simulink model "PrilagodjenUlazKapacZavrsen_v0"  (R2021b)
settings: Solver=VariableStepAuto  StartTime=0.0  StopTime=200e-09  MaxStep=0.1e-09  RelTol=1e-3
libraries: fl_lib x9, nesl_utility x5, simulink x1, ee_lib x1

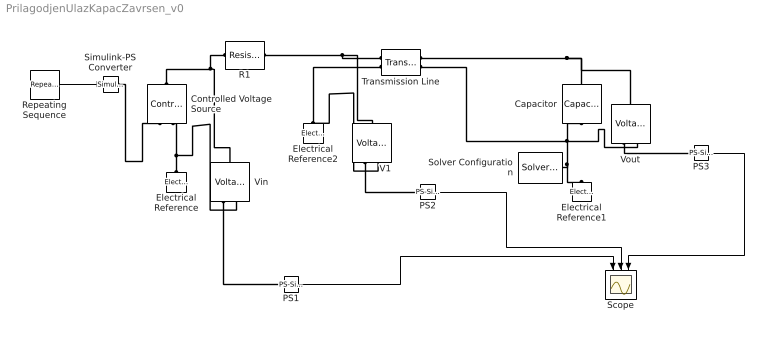
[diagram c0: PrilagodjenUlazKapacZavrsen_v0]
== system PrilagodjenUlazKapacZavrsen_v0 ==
  Capacitor : fl_lib/Electrical/Electrical Elements/Capacitor  c=200 pF  r=1e-6 Ohm  g=0 1/Ohm  i_specify=off  i_priority=None  i=0 A  i_nominal_specify=off  i_nominal_unit=A  i_nominal_value=1  v_specify=off  v_priority=None  v=0 V  v_nominal_specify=off  v_nominal_unit=V  v_nominal_value=1  vc_specify=off  vc_priority=High  vc=0 V  vc_nominal_specify=off  vc_nominal_unit=V  vc_nominal_value=1
  Controlled Voltage Source : fl_lib/Electrical/Electrical Sources/Controlled Voltage Source
  Electrical Reference : fl_lib/Electrical/Electrical Elements/Electrical Reference
  Electrical Reference1 : fl_lib/Electrical/Electrical Elements/Electrical Reference
  Electrical Reference2 : fl_lib/Electrical/Electrical Elements/Electrical Reference
  PS1 : nesl_utility/PS-Simulink Converter  PhysicalDomain=network_engine_domain  SubClassName=ps_output  LeftPortType=input  RightPortType=output  PseudoPeriodic=off  Frequencies=[]  Unit=inherit  AffineConversion=off
  PS2 : nesl_utility/PS-Simulink Converter  PhysicalDomain=network_engine_domain  SubClassName=ps_output  LeftPortType=input  RightPortType=output  PseudoPeriodic=off  Frequencies=[]  Unit=inherit  AffineConversion=off
  PS3 : nesl_utility/PS-Simulink Converter  PhysicalDomain=network_engine_domain  SubClassName=ps_output  LeftPortType=input  RightPortType=output  PseudoPeriodic=off  Frequencies=[]  Unit=inherit  AffineConversion=off
  R1 : fl_lib/Electrical/Electrical Elements/Resistor  R=50 Ohm  i_specify=off  i_priority=None  i=0 A  i_nominal_specify=off  i_nominal_unit=A  i_nominal_value=1  v_specify=off  v_priority=None  v=0 V  v_nominal_specify=off  v_nominal_unit=V  v_nominal_value=1
  Repeating Sequence : simulink/Sources/Repeating Sequence  rep_seq_t=[0 1 20 21 300]*1e-9  rep_seq_y=[0 1 1 0 0]
  Scope : Scope  NumInputPorts=3
  Simulink-PS Converter : nesl_utility/Simulink-PS Converter  PhysicalDomain=network_engine_domain  SubClassName=ps_input  LeftPortType=input  RightPortType=output  PseudoPeriodic=off  Frequencies=[]  NoiseDistribution=none  NoiseParameters=[]  Unit=1  AffineConversion=off  FilteringAndDerivatives=provide  SimscapeFilterOrder=1  InputFilterTimeConstant=0.001  UdotUserProvided=0
  Solver Configuration : nesl_utility/Solver Configuration  PhysicalDomain=network_engine_domain  SubClassName=solver  LeftPortType=input  RightPortType=generic  Tones=[]  Harmonics=[]  SimulateNoise=off  Profile=off  UseLocalSampling=off  EnableSwitchedLinearOptims=on  FrequencyDomain=off  UseCCode=off  RelTol=0.001  AbsTol=1e-06  MinStep=1e-09  ToWorkspace=off  RevertToSquareIcSolve=off  NumHomotopyIterations=100  PhasorMode=off  PhasorModeNumHarmonics=1  DoDC=off  ResidualTolerance=1e-09  UseLocalSolver=off  LocalSolverChoice=NE_BACKWARD_EULER_ADVANCER  LocalSolverSampleTime=0.001  DoFixedCost=off  MaxNonlinIter=3  MaxModeIter=2  ComputeImpulses=off  ImpulseIterations=2  LinearAlgebra=auto  EquationFormulation=NE_TIME_EF  DelaysMemoryBudget=1024  AutomaticFiltering=on  FilteringTimeConstant=0.001  PartitionStorageMethod=AS_NEEDED  PartitionMemoryBudget=1024  PartitionMethod=ROBUST
  Transmission Line : ee_lib/Passive/Lines/Transmission Line  model_type=1  TD=60 ns  LC_param=1  Z0_delay_based=50 Ohm  Z0=50 Ohm  freq=60 Hz  Ll=220 uH/m  L=220 uH/m  C=90 pF/m  R=0.3 Ohm/m  G=5e-6 S/m  LEN=1 m  N=1
  V1 : fl_lib/Electrical/Electrical Sensors/Voltage Sensor
  Vin : fl_lib/Electrical/Electrical Sensors/Voltage Sensor
  Vout : fl_lib/Electrical/Electrical Sensors/Voltage Sensor
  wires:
  Repeating Sequence/1 -> Simulink-PS Converter/1
  PS1/1 -> Scope/1
  PS2/1 -> Scope/2
  PS3/1 -> Scope/3
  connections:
  Electrical Reference2/LConn1 -- V1/RConn2 -- Transmission Line/LConn2
  Transmission Line/RConn2 -- Capacitor/RConn1 -- Vout/RConn2 -- Solver Configuration/RConn1 -- Electrical Reference1/LConn1
  Electrical Reference/LConn1 -- Vin/RConn2 -- Controlled Voltage Source/RConn2
  Controlled Voltage Source/LConn1 -- Vin/LConn1 -- R1/LConn1
  R1/RConn1 -- V1/LConn1 -- Transmission Line/LConn1
  Transmission Line/RConn1 -- Capacitor/LConn1 -- Vout/LConn1
  Simulink-PS Converter/RConn1 -- Controlled Voltage Source/RConn1
  Vout/RConn1 -- PS3/LConn1
  V1/RConn1 -- PS2/LConn1
  Vin/RConn1 -- PS1/LConn1
